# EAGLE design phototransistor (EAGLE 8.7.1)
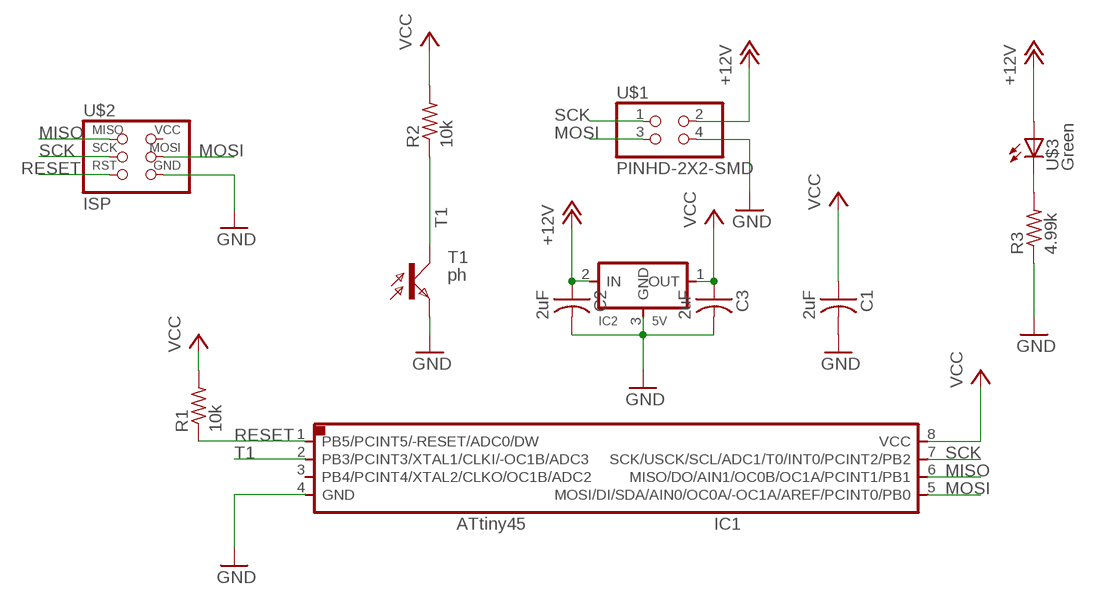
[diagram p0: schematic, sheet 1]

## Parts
C1  2uF  CAP-US1206FAB  [C1206FAB]
C2  2uF  CAP-US1206FAB  [C1206FAB]
C3  2uF  CAP-US1206FAB  [C1206FAB]
IC1  T45  ATTINY45SI  [SOIC8]
IC2  5V  REGULATORSOT23  [SOT23]
R1  10k  RES-US1206FAB  [R1206FAB]
R2  10k  RES-US1206FAB  [R1206FAB]
R3  4.99k  RES-US1206FAB  [R1206FAB]
T1  ph  PHOTOTRANSISTOR-NPN1206  [OP1206]
U$1  PINHD-2X2-SMD  [2X02SMD]
U$2  ISP  AVRISPSMD  [2X03SMD]
U$3  Green  LEDFAB1206  [LED1206FAB]

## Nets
+12V: C2.1 IC2.2(IN) U$1.2 U$3.1(A)
GND: C1.2 C2.2 C3.2 IC1.4(GND) IC2.3(GND) R3.1 T1.EMITTER(E) U$1.4 U$2.6(GND)
MISO: IC1.6(MISO/DO/AIN1/OC0B/OC1A/PCINT1/PB1) U$2.1(MISO)
MOSI: IC1.5(MOSI/DI/SDA/AIN0/OC0A/-OC1A/AREF/PCINT0/PB0) U$1.3 U$2.4(MOSI)
N$1: R3.2 U$3.2(C)
RESET: IC1.1(PB5/PCINT5/-RESET/ADC0/DW) R1.1 U$2.5(RST)
SCK: IC1.7(SCK/USCK/SCL/ADC1/T0/INT0/PCINT2/PB2) U$1.1 U$2.3(SCK)
T1: IC1.2(PB3/PCINT3/XTAL1/CLKI/-OC1B/ADC3) R2.1 T1.COLLECTOR(C)
VCC: C1.1 C3.1 IC1.8(VCC) IC2.1(OUT) R1.2 R2.2
Unconnected: IC1.3(PB4/PCINT4/XTAL2/CLKO/OC1B/ADC2) U$2.2(VCC)

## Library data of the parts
C1-C3 = fab.lbr:CAP-US
IC1 = fab.lbr:ATTINY45
IC2 = fab:REGULATOR
R1 R2 = fab.lbr:RES-US: Resistor (US Symbol)
R3 = fab:RES-US: Resistor (US Symbol)
T1 = fab.lbr:PHOTOTRANSISTOR-NPN
U$1 = fab:PINHD-2X2-SMD
U$2 = fab.lbr:AVRISP
U$3 = fab:LED: LED

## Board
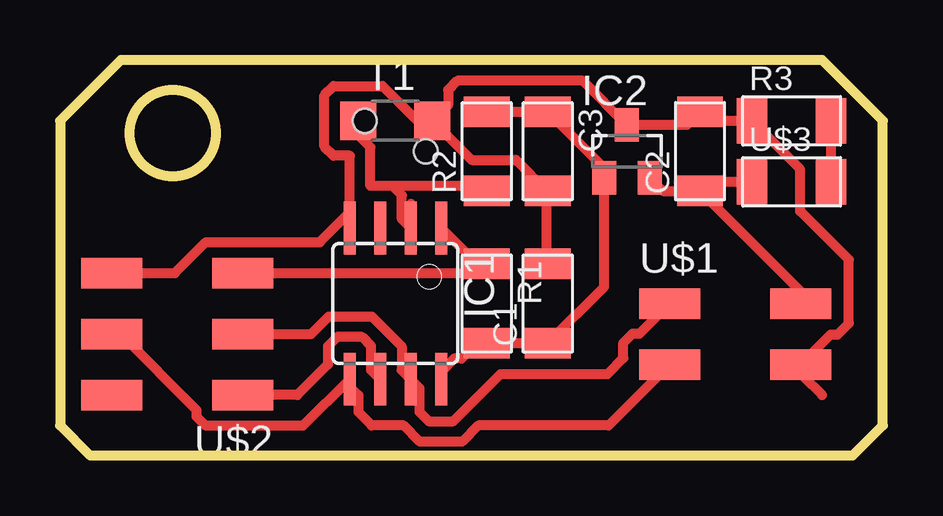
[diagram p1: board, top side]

Size 34.29 x 16.51 mm. Coordinates in mm from the lower left corner, seen from the top.
Outline: 34.29,1.27 34.29,13.97 31.75,16.51 2.54,16.51 0,13.97 0,1.27 1.27,0 33.02,0 34.29,1.27
Outline: circle at 4.7,13.46 radius 1.8
Copper layers 1: Top 0.035mm
Design rules "basbasic": minimum track width 0.3mm, minimum drill 0.9mm, track to track 0.45mm, track to pad 0.45mm, pad to pad 0.45mm, via to via 0.45mm, smd to smd 6mil, copper to edge 40mil, drill to drill 6mil, minimum pad ring 10mil, minimum via ring 8mil, stop-mask expansion 4mil, vias tented up to drill 0mil, thermal gap 10mil
Holes 1 mm at 12.7,13.97 15.24,12.7

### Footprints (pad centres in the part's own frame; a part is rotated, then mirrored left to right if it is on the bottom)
C1206FAB = smd 1.27 x 1.905: 1 -1.651,0; 2 1.651,0
SOIC8 = smd 0.5 x 2.2: 1 -1.905,-3.154; 2 -0.645,-3.154; 3 0.625,-3.154; 4 1.895,-3.154; 5 1.905,3.154; 6 0.635,3.154; 7 -0.635,3.154; 8 -1.905,3.154
SOT23 = smd 1 x 1.4: 1 -0.95,-1.1; 2 0.95,-1.1; 3 0,1.1
R1206FAB = smd 1.27 x 1.905: 1 -1.651,0; 2 1.651,0
OP1206 = smd 1.5 x 1.6: COLLECTOR -1.55,0; EMITTER 1.55,0
2X02SMD = smd 2.54 x 1.27: 1 -2.54,1.27; 2 2.92,1.27; 3 -2.54,-1.27; 4 2.92,-1.27
2X03SMD = smd 2.54 x 1.27: 1 -2.54,2.54; 2 2.92,2.54; 3 -2.54,0; 4 2.92,0; 5 -2.54,-2.54; 6 2.92,-2.54
LED1206FAB = smd 1.27 x 1.905: 1 -1.651,0; 2 1.651,0

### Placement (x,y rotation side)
C1  20.32,6.35 90 top
C2  26.67,12.7 90 top
C3  20.32,12.7 270 top
IC1  13.97,6.35 180 top
IC2  23.62,12.7 0 top
R1  17.78,6.35 270 top
R2  17.78,12.7 90 top
R3  30.48,13.97 0 top
T1  13.97,13.97 0 top
U$1  27.94,5.08 0 top
U$2  5.08,5.08 180 top
U$3  30.48,11.43 0 top

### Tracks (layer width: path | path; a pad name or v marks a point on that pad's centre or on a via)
+12V
  Top 0.406: C2.1 25.78,11.43 U$3.1 | IC2.2 25.12,11.05 C2.1 | C2.1 30.86,6.86 U$1.2
GND
  Top 0.406: 20.83,8 C1.2 20.29,8.03 20.29,11.05 | T1.EMITTER 17.15,12.34 19,12.34 20.29,11.05 | 20.29,11.05 C3.2 | IC1.4 12.07,10.16 | 12.07,10.16 12.07,12.52 11.4,12.52 11.02,12.9 11.02,15.04 11.4,15.42 13.44,15.42 14.89,13.97 T1.EMITTER | T1.EMITTER 16.17,14.62 16.17,15.26 16.56,15.64 21.78,15.64 IC2.3 26.12,13.8 C2.2 27.05,13.97 R3.1 30.84,11.96 30.84,10.21 32.87,8.18 32.87,5.53 32.4,5.06 32.11,5.06 U$1.4 30.86,3.56 arc45 30.95,3.34 31.75,2.54 | U$2.6 4.79,7.62 6.08,8.91 10.82,8.91 12.07,10.16
MISO
  Top 0.406: IC1.6 12.97,3.56 12.97,4.57 12.59,4.95 11.54,4.95 11.16,4.57 11.16,3.81 9.89,2.54 U$2.1
MOSI
  Top 0.406: U$1.3 22.86,1.27 17.43,1.27 16.75,0.59 15,0.59 14.32,1.27 12.99,1.27 12.43,1.83 12.43,2.52 12.11,2.84 12.11,3.15 IC1.5 10.12,1.25 6.08,1.25 5.7,1.63 5.7,1.91 2.52,5.08 U$2.4
N$1
  Top 0.406: U$3.2 R3.2
RESET
  Top 0.406: IC1.1 17.38,8 R1.1 17.4,7.62 U$2.5
SCK
  Top 0.406: U$1.1 24.15,5.1 23.86,5.1 23.48,4.72 23.48,4.08 22.81,3.41 18.36,3.41 16.4,1.44 15.35,1.44 14.97,1.83 14.97,2.83 IC1.7 14.24,3.56 14.24,4.57 13,5.81 11.19,5.81 10.46,5.08 U$2.3
T1
  Top 0.406: 14.62,10.51 IC1.2 14.25,9.87 14.25,10.88 13.87,11.26 | R2.1 17.57,11.26 13.87,11.26 | 13.87,11.26 12.93,11.26 12.93,12.87 12.42,13.38 T1.COLLECTOR
VCC
  Top 0.406: IC1.8 15.92,3.24 15.92,3.55 16.42,4.05 16.73,4.05 17.38,4.7 R1.2 C1.1 22.67,7.05 IC2.1 22.67,12 C3.1 R2.2

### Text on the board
203bmp: G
